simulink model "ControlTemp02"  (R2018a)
settings: Solver=VariableStepAuto  StartTime=0.0  StopTime=2  RelTol=1e-3
undefined symbols (not defined in the file): be70, ControlTemp02, sdiscope

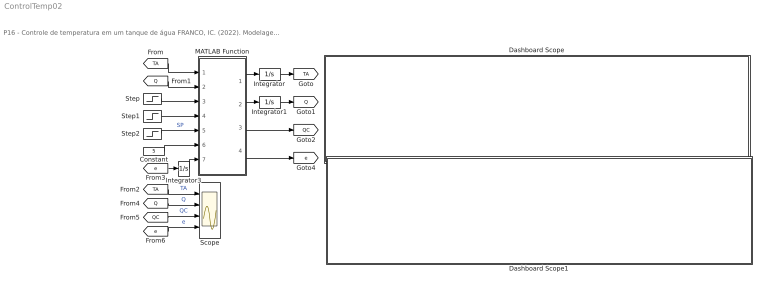
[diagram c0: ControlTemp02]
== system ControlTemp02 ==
  note: P16 - Controle de temperatura em um tanque de água FRANCO, IC. (2022). Modelagem e Simulação: Problemas Típicos da Engenharia Química para Simulação e Análise. NOTAS DE AULA INOVADORAS. The Journal of Engineering and Exact Sciences. Material Complementar.
  Constant : Constant  Value=5
  Dashboard Scope : Subsystem  DialogController=hmiCreateDDGDialog  IsWebBlock=on  mask(MWDashboardBlock){webBlockId=228661cc-797c-493c-88b7-9a33a8523ab2, webBlockType=sdiscope, ShowInitialText=on, HMISrcModelName=ControlTemp02}
      mask prompts: webBlockId "WebBlock Id"; webBlockType "WebBlock Type"; HMISrcModelName "Source Model"
      mask help: SimulinkHMI:dialogs:HMIScopeDialogDesc
  Dashboard Scope1 : Subsystem  DialogController=hmiCreateDDGDialog  IsWebBlock=on  mask(MWDashboardBlock){webBlockId=019602e2-2ca1-4a06-be70-3c4b76dd941d, webBlockType=sdiscope, ShowInitialText=on, HMISrcModelName=ControlTemp02}
      mask prompts: webBlockId "WebBlock Id"; webBlockType "WebBlock Type"; HMISrcModelName "Source Model"
      mask help: SimulinkHMI:dialogs:HMIScopeDialogDesc
  Integrator : Integrator  InitialCondition=20
  Integrator1 : Integrator  InitialCondition=6
  Integrator3 : Integrator
  MATLAB Function : MATLAB Function  TreatAsAtomicUnit=on
  Scope : Scope  NumInputPorts=4
  Step : Step  Time=0  Before=20  After=20  SampleTime=0
  Step1 : Step  Time=0  Before=600  After=600  SampleTime=0
  Step2 : Step  Time=0  Before=80  After=80  SampleTime=0
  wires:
  [TA] -> MATLAB Function/1(TA)
  MATLAB Function/4(e) -> [e]
  [e] -> Integrator3/1
  [Q] -> MATLAB Function/2(Q)
  Integrator/1 -> [TA]
  MATLAB Function/2(dQ) -> Integrator1/1
  Integrator3/1 -> MATLAB Function/7(ie)
  MATLAB Function/1(dTA) -> Integrator/1
  Integrator1/1 -> [Q]
  Step/1 -> MATLAB Function/3(T0)
  Step1/1 -> MATLAB Function/4(F)
  Constant/1 -> MATLAB Function/6(KC)
  MATLAB Function/3(QC) -> [QC]
  [TA] -> Scope/1  "TA"
  [Q] -> Scope/2  "Q"
  [QC] -> Scope/3  "QC"
  [e] -> Scope/4  "e"
  Step2/1 -> MATLAB Function/5(Tsp)  "SP"

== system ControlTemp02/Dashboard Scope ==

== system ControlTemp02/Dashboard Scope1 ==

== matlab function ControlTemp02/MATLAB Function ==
function [dTA,dQ,QC,e] = fcn(TA,Q,T0,F,Tsp,KC,ie)
%parâmetros
Cp   =   1.0;
Q0   = 300.0;
V    = 100.0;
rho  =   1.0;
tauQ =   0.05;

%% controlador PI
%parâmetros do controlador
taui =   0.1;
%error
e=Tsp-TA;
%variável manipulada
QC=Q0+KC*e+(KC/taui)*ie;

%modelo matemático
dTA = (F/V)*(T0-TA)+Q;
dQ  = (QC-Q)/tauQ;
end
